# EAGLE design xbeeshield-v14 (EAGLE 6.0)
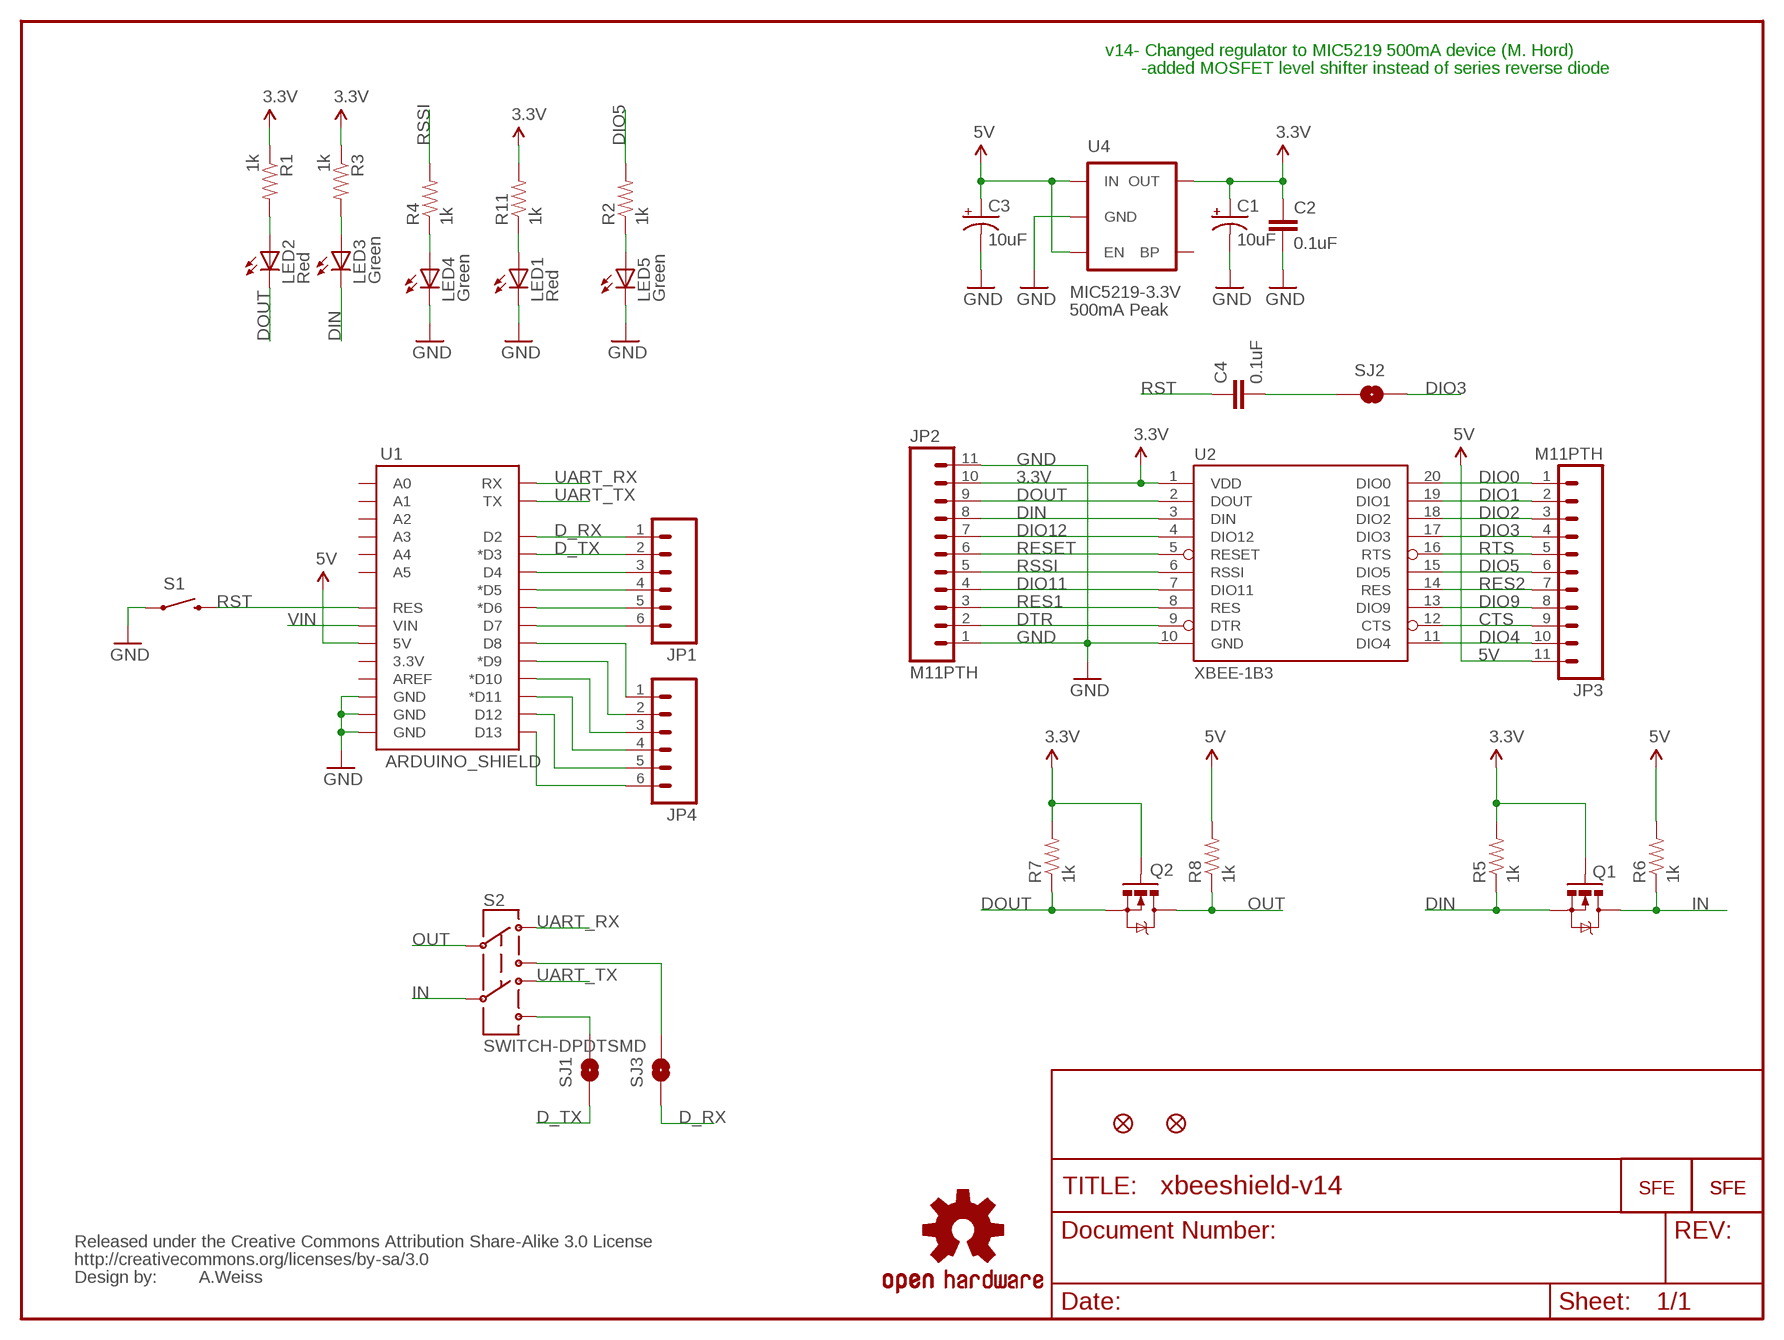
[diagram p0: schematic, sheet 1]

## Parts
C1  10uF  CAP_POL1206  [EIA3216]
C2  0.1uF  CAP0402-CAP  [0402-CAP]
C3  10uF  CAP_POL1206  [EIA3216]
C4  0.1uF  CAP0402-CAP  [0402-CAP]
JP1  M06SIP  [1X06]
JP2  M11PTH  [1X11]
JP3  M11PTH  [1X11]
JP4  M06SIP  [1X06]
JP5  FIDUCIAL1X2  [FIDUCIAL-1X2]
JP6  FIDUCIAL1X2  [FIDUCIAL-1X2]
JP7  LOGO-SFENEW  [SFE-NEW-WEBLOGO]
LED1  Red  LED0603  [LED-0603]
LED2  Red  LED0603  [LED-0603]
LED3  Green  LED0603  [LED-0603]
LED4  Green  LED0603  [LED-0603]
LED5  Green  LED0603  [LED-0603]
Q1  MOSFET-NCHANNELSMD  [SOT23-3]
Q2  MOSFET-NCHANNELSMD  [SOT23-3]
R1  1k  RESISTOR0402-RES  [0402-RES]
R2  1k  RESISTOR0402-RES  [0402-RES]
R3  1k  RESISTOR0402-RES  [0402-RES]
R4  1k  RESISTOR0402-RES  [0402-RES]
R5  1k  RESISTOR0402-RES  [0402-RES]
R6  1k  RESISTOR0402-RES  [0402-RES]
R7  1k  RESISTOR0402-RES  [0402-RES]
R8  1k  RESISTOR0402-RES  [0402-RES]
R11  1k  RESISTOR0402-RES  [0402-RES]
S1  SWITCH-MOMENTARY-2SMD  [TACTILE_SWITCH_SMD]
S2  SWITCH-DPDTSMD  [AYZ0202]
SJ1  D_TX  SOLDERJUMPERNC  [SJ_2S]
SJ2  SOLDERJUMPERTRACE  [SJ_2S-TRACE]
SJ3  D_RX  SOLDERJUMPERNC  [SJ_2S]
U1  ARDUINO_SHIELD  ARDUINO_SHIELDLABEL  [DUEMILANOVE_SHIELD]
U2  XBEE-1B3  [XBEE-SMD]
U4  V_REG_LDOSMD  [SOT23-5]
U$1  LOGO-SFESK  [SFE-LOGO-FLAME]
U$4  LOGO-SFENEW  [SFE-NEW-WEBLOGO]
U$5  CREATIVE_COMMONS  [CREATIVE_COMMONS]
U$8  OSHW-LOGOS  [OSHW-LOGO-S]

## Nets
3.3V: C1.A(+) C2.1 JP2.10 Q1.1(G) Q2.1(G) R1.1 R3.1 R5.2 R7.2 R11.2 U2.1(VDD) U4.5(OUT)
5V: C3.A(+) JP3.11 R6.2 R8.2 U1.5V U4.1(IN) U4.3(EN)
CTS: JP3.9 U2.12(CTS)
D_RX: JP1.1 SJ3.1 U1.D2
D_TX: JP1.2 SJ1.1 U1.D3(*D3)
DIN: JP2.8 LED3.C Q1.2(S) R5.1 U2.3(DIN)
DIO0: JP3.1 U2.20(DIO0)
DIO1: JP3.2 U2.19(DIO1)
DIO2: JP3.3 U2.18(DIO2)
DIO3: JP3.4 SJ2.2 U2.17(DIO3)
DIO4: JP3.10 U2.11(DIO4)
DIO5: JP3.6 R2.2 U2.15(DIO5)
DIO9: JP3.8 U2.13(DIO9)
DIO11: JP2.4 U2.7(DIO11)
DIO12: JP2.7 U2.4(DIO12)
DOUT: JP2.9 LED2.C Q2.2(S) R7.1 U2.2(DOUT)
DTR: JP2.2 U2.9(DTR)
GND: C1.C(-) C2.2 C3.C(-) JP2.1 JP2.11 LED1.C LED4.C LED5.C S1.1 U1.GND@0(GND) U1.GND@1(GND) U1.GND@2(GND) U2.10(GND) U4.2(GND)
IN: Q1.3(D) R6.1 S2.5
N$1: LED2.A R1.2
N$2: LED4.A R4.1
N$4: LED3.A R3.2
N$5: C4.2 SJ2.1
N$17: JP4.1 U1.D8
N$18: JP4.2 U1.D9(*D9)
N$30: JP4.3 U1.D10(*D10)
N$38: LED1.A R11.1
N$43: JP4.4 U1.D11(*D11)
N$55: JP4.5 U1.D12
N$67: JP4.6 U1.D13
N$139: LED5.A R2.1
N$140: S2.6 SJ1.2
N$141: S2.3 SJ3.2
N$142: JP1.3 U1.D4
N$143: JP1.4 U1.D5(*D5)
N$144: JP1.5 U1.D6(*D6)
N$145: JP1.6 U1.D7
OUT: Q2.3(D) R8.1 S2.2
RES1: JP2.3 U2.8(RES)
RES2: JP3.7 U2.14(RES)
RESET: JP2.6 U2.5(RESET)
RSSI: JP2.5 R4.2 U2.6(RSSI)
RST: C4.1 S1.3 U1.RES
RTS: JP3.5 U2.16(RTS)
UART_RX: S2.1 U1.RX
UART_TX: S2.4 U1.TX
VIN: U1.VIN
Unconnected: U1.3.3V U1.A0 U1.A1 U1.A2 U1.A3 U1.A4 U1.A5 U1.AREF U4.4(BP)

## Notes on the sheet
- v14- Changed regulator to MIC5219 500mA device (M. Hord)
- -added MOSFET level shifter instead of series reverse diode
- MIC5219-3.3V
- 500mA Peak
- A.Weiss

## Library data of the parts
C1 C3 = SparkFun:CAP_POL: Capacitor Polarized
C2 C4 = SparkFun:CAP: Capacitor
JP1 JP4 = SparkFun:M06: Header 6 Standard 6-pin 0.1" header. Use with straight break away headers (SKU : PRT-00116), right angle break away headers (PRT-00553), swiss pins (PRT-00743), machine pins (PRT-00117), and female headers (PRT-00115). Molex polarized connector foot print use with SKU : PRT-08094 with associated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
JP2 JP3 = SparkFun:M11: Header 11 Standard 11-pin 0.1" header. Use with straight break away headers (SKU : PRT-00116), right angle break away headers (PRT-00553), swiss pins (PRT-00743), machine pins (PRT-00117), and female headers (PRT-00115).
JP5 JP6 = SparkFun:FIDUCIAL: Fiducial Alignment Points
JP7 = SparkFun-Aesthetics:LOGO-SFE: Spark Fun Electronics PCB Logo
LED1-LED5 = SparkFun:LED: LEDs
Q1 Q2 = SparkFun-DiscreteSemi:MOSFET-NCHANNEL: Generic NMOS footprint
R1-R8 R11 = SparkFun:RESISTOR: Resistor
S1 = SparkFun:SWITCH-MOMENTARY-2
S2 = SparkFun:SWITCH-DPDT: DPDT Version of the COM-00597
SJ1-SJ3 = SparkFun:SOLDERJUMPER: Solder Jumper
U1 = SparkFun:ARDUINO_SHIELD
U2 = SparkFun:XBEE-1
U4 = SparkFun-PowerIC:V_REG_LDO: Voltage Regulator LDO Standard 150mA LDO voltage regulator in SOT-23 layout. Micrel part MIC5205. BP (by-pass) pin is used to lower output noise with 470pF cap.
U$1 U$4 = SparkFun:LOGO-SFE: Spark Fun Electronics PCB Logo
U$5 = SparkFun:CREATIVE_COMMONS
U$8 = SparkFun-Aesthetics:OSHW-LOGO: Open Source Hardware Logo This logo indicates the piece of hardware it is found on incorporates a OSHW license and/or adheres to the definition of open source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

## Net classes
0 default: width 0.203 mm
1 vcc: width 0.305 mm

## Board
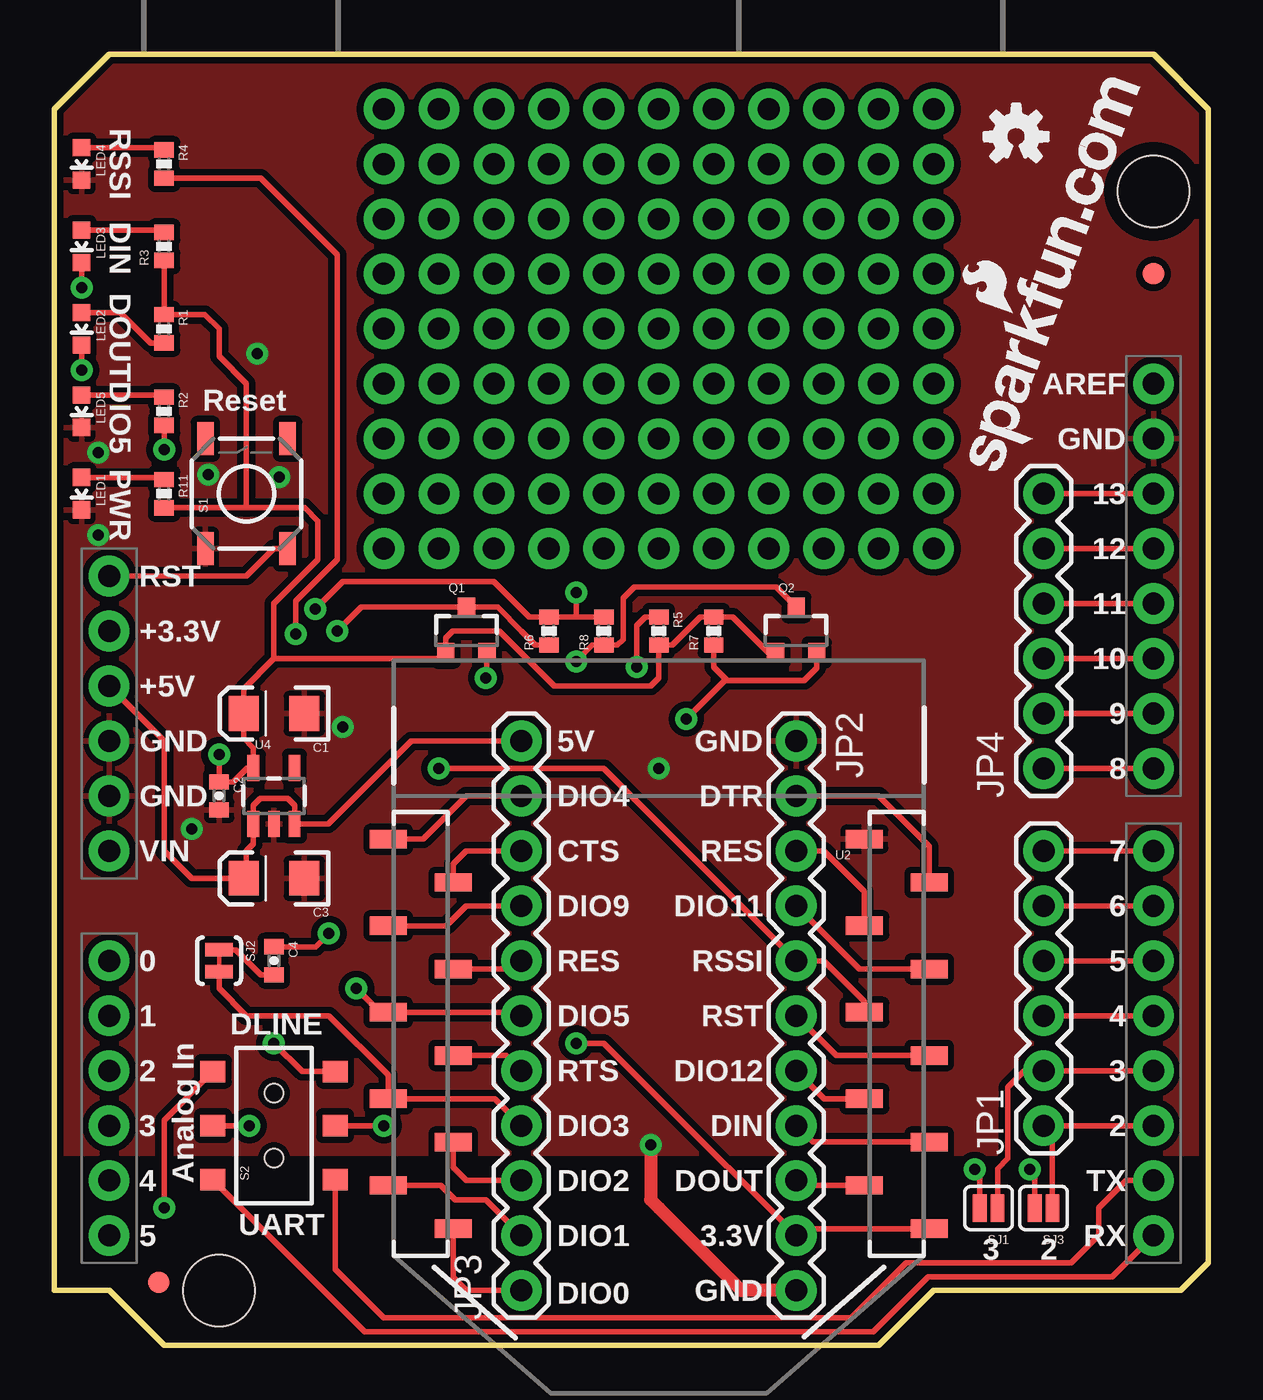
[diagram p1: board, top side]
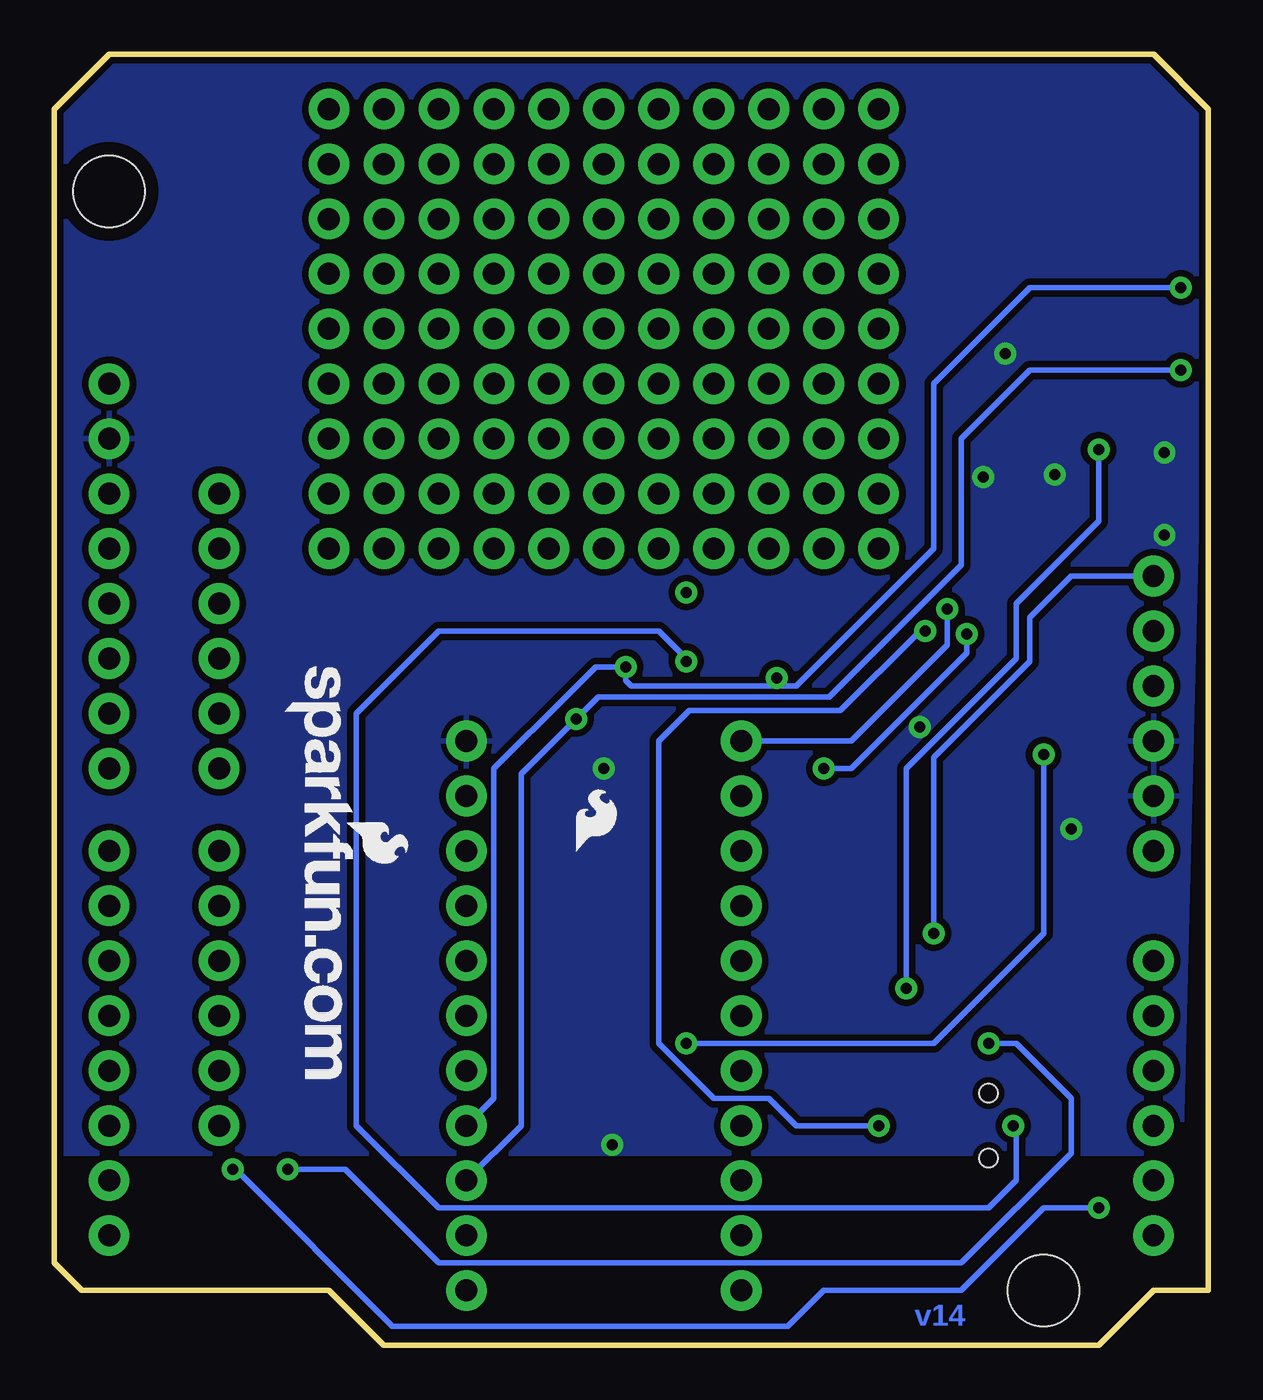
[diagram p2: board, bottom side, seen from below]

Size 53.34 x 59.69 mm. Coordinates in mm from the lower left corner, seen from the top.
Outline: 0,2.54 0,57.15 2.54,59.69 50.8,59.69 53.34,57.15 53.34,3.81 52.07,2.54 40.64,2.54 38.1,0 5.08,0 2.54,2.54 0,2.54
Copper layers (1*16): Top 0.035mm / dielectric 1.5mm / Bottom 0.035mm
Design rules: minimum track width 8mil, minimum drill 20mil, track to track 8mil, track to pad 8mil, pad to pad 8mil, via to via 8mil, smd to smd 8mil, copper to edge 8mil, drill to drill 8mil, minimum pad ring 12mil, minimum via ring 10mil, stop-mask expansion 4mil, vias tented up to drill 20mil, thermal gap 10mil

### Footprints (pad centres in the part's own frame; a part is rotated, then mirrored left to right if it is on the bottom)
EIA3216 = smd 1.4 x 1.6: A 1.4,0; C -1.4,0
0402-CAP = smd 0.7 x 0.9: 1 -0.65,0; 2 0.65,0
1X06 = drill 1.016 pad 1.88: 1 0,0; 2 2.54,0; 3 5.08,0; 4 7.62,0; 5 10.16,0; 6 12.7,0
1X11 = drill 1.016 pad 1.88: 1 0,0; 2 2.54,0; 3 5.08,0; 4 7.62,0; 5 10.16,0; 6 12.7,0; 7 15.24,0; 8 17.78,0; 9 20.32,0; 10 22.86,0; 11 25.4,0
FIDUCIAL-1X2 = smd 1 x 1: 1 0,0
LED-0603 = smd 0.8 x 0.8: A 0,-0.75; C 0,0.75
SOT23-3 = smd 0.8 x 0.9: 1 -0.95,-1; 2 0.95,-1; 3 0,1.1
0402-RES = smd 0.7 x 0.9: 1 -0.65,0; 2 0.65,0
TACTILE_SWITCH_SMD = smd 1.524 x 0.762: 1 -2.54,1.905; 2 2.54,1.905; 3 -2.54,-1.905; 4 2.54,-1.905
AYZ0202 = smd 1 x 1.15: 1 -2.5,2.825; 2 0,2.825; 3 2.5,2.825; 4 -2.5,-2.825; 5 0,-2.825; 6 2.5,-2.825 | hole 0.85: 1.5,0; -1.5,0
SJ_2S = smd 0.635 x 1.27: 1 -0.412,0; 2 0.412,0
SJ_2S-TRACE = smd 0.635 x 1.27: 1 -0.508,0; 2 0.508,0
DUEMILANOVE_SHIELD = drill 1.016 pad 1.88: 3.3V 50.8,26.67; 5V 50.8,29.21; A0 50.8,41.91; A1 50.8,44.45; A2 50.8,46.99; A3 50.8,49.53; A4 50.8,52.07; A5 50.8,54.61; AREF 2.54,15.24; D2 2.54,49.53; D3 2.54,46.99; D4 2.54,44.45; D5 2.54,41.91; D6 2.54,39.37; D7 2.54,36.83; D8 2.54,33.02; D9 2.54,30.48; D10 2.54,27.94; D11 2.54,25.4; D12 2.54,22.86; D13 2.54,20.32; GND@0 50.8,31.75; GND@1 50.8,34.29; GND@2 2.54,17.78; RES 50.8,24.13; RX 2.54,54.61; TX 2.54,52.07; VIN 50.8,36.83 | hole 3.302: 45.72,57.15; 2.54,6.35
XBEE-SMD = smd 1.7 x 0.85: 1 -12.5,20; 2 -9.5,18; 3 -12.5,16; 4 -9.5,14; 5 -12.5,12; 6 -9.5,10; 7 -12.5,8; 8 -9.5,6; 9 -12.5,4; 10 -9.5,2; 11 12.5,2; 12 9.5,4; 13 12.5,6; 14 9.5,8; 15 12.5,10; 16 9.5,12; 17 12.5,14; 18 9.5,16; 19 12.5,18; 20 9.5,20
SOT23-5 = smd 0.55 x 1.2: 1 -0.95,-1.3; 2 0,-1.3; 3 0.95,-1.3; 4 0.95,1.3; 5 -0.95,1.3

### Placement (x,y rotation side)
C1  10.16,29.21 180 top
C2  7.62,25.4 270 top
C3  10.16,21.59 180 top
C4  10.16,17.78 270 top
JP1  45.72,10.16 90 top
JP2  34.29,27.94 270 top
JP3  21.59,2.54 90 top
JP4  45.72,26.67 90 top
JP5  4.83,2.92 0 top
JP6  50.8,49.53 0 top
JP7  42.67,31.37 270 bottom
LED1  1.27,39.37 180 top
LED2  1.27,46.99 180 top
LED3  1.27,50.8 180 top
LED4  1.27,54.61 180 top
LED5  1.27,43.18 180 top
Q1  19.05,33.02 0 top
Q2  34.29,33.02 0 top
R1  5.08,46.99 270 top
R2  5.08,43.18 270 top
R3  5.08,50.8 90 top
R4  5.08,54.61 270 top
R5  27.94,33.02 270 top
R6  22.86,33.02 90 top
R7  30.48,33.02 90 top
R8  25.4,33.02 90 top
R11  5.08,39.37 270 top
S1  8.89,39.37 90 top
S2  10.16,10.16 90 top
SJ1  43.18,6.35 180 top
SJ2  7.62,17.78 270 top
SJ3  45.72,6.35 180 top
U1  53.34,59.69 180 top
U2  27.94,25.4 180 top
U4  10.16,25.4 0 top
U$1  29.21,22.86 0 bottom
U$4  44.54,39.97 70 top
U$5  not placed on the board
U$8  44.45,55.88 0 top

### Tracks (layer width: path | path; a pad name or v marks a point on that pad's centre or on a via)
3.3V  (via drill 0.51)
  Top 0.254: R3.1 R1.1 6.97,47.64 7.62,46.99 7.62,45.72 8.89,44.45 8.89,40.64 8.89,38.72 | U2.1 34.61,5.4 JP2.10 27.94,11.43 25.4,13.97 v24.13,13.97 | 10.16,31.75 8.76,30.35 C1.A 8.76,28.07 9.21,27.62 U4.5 8.92,26.7 8.27,26.05 C2.1 v7.62,27.3 | Q2.1 33,32.02 32,33.02 31.35,33.67 R7.2 29.86,33.67 29.21,33.02 28.56,32.37 R5.2 27.94,30.86 27.56,30.48 23.11,30.48 20.57,33.02 18.41,33.02 18.16,32.77 18.1,32.7 Q1.1 17.83,31.75 10.16,31.75 | R11.2 6.97,38.72 8.89,38.72 | 8.89,38.72 11.57,38.72 12.19,38.1 12.19,36.32 10.16,34.29 10.16,31.75
  Bottom 0.254: v24.13,13.97 12.7,13.97 7.62,19.05 v7.62,27.3
5V  (via drill 0.51)
  Top 0.254: U1.5V 5.08,27.94 5.08,22.86 6.35,21.59 C3.A 8.89,21.72 8.89,22.86 9.21,23.18 U4.1 9.21,24.96 9.53,25.27 10.79,25.27 11.11,24.96 U4.3 12.67,24.1 16.51,27.94 JP3.11 | 24.13,33.67 R6.2 21.96,33.67 20.32,35.31 14.1,35.31 13.34,35.31 v12.06,34.04 | 24.13,33.67 R8.2 | v24.13,34.8 24.13,33.67
  Bottom 0.254: JP3.11 16.51,27.94 12.7,31.75 12.06,32.38 v12.06,34.04
CTS
  Top 0.254: U2.12 18.44,22.25 19.05,22.86 JP3.9
D_RX
  Top 0.254: U1.D2 JP1.1 46.13,9.75 SJ3.1
D_TX
  Top 0.254: U1.D3 JP1.2 44.83,12.7 44.07,11.94 44.07,8.64 43.59,8.16 SJ1.1
DIN  (via drill 0.51)
  Top 0.254: v1.27,48.9 LED3.C | R5.1 27.32,33.67 26.92,33.27 v26.92,31.37 | Q1.2 20,30.92 v19.94,30.86 | U2.3 35.05,9.4 JP2.8
  Bottom 0.254: v1.27,48.9 3.17,48.9 8.26,48.9 12.7,44.45 12.7,40.64 12.7,38.1 12.7,36.83 19.05,30.48 19.94,30.48 | JP2.8 33.02,11.43 33.02,26.67 29.59,30.1 28.32,31.37 v26.92,31.37 26.92,30.73 26.67,30.48 19.94,30.48 | v19.94,30.86 19.94,30.48
DIO0
  Top 0.254: U2.20 18.44,3.15 19.05,2.54 JP3.1
DIO1
  Top 0.254: JP3.2 19.94,6.73 18.54,6.73 17.87,7.4 U2.19
DIO2
  Top 0.254: U2.18 18.44,8.23 19.05,7.62 JP3.3
DIO3
  Top 0.254: JP3.4 20.35,11.4 U2.17 15.44,12.5 12.7,15.24 8.89,15.24 7.62,16.51 SJ2.2
DIO4
  Top 0.254: U2.11 17.05,23.4 19.05,25.4 JP3.10
DIO5  (via drill 0.51)
  Top 0.254: v5.08,41.4 R2.2 | JP3.6 21.43,15.4 U2.15 15.08,15.4 v13.97,16.51
  Bottom 0.254: v13.97,16.51 13.97,25.4 13.97,26.67 8.89,31.75 8.89,34.29 5.08,38.1 v5.08,41.4
DIO9
  Top 0.254: U2.13 18.13,19.4 19.05,20.32 JP3.8
DIO11
  Top 0.254: U2.7 37.21,17.4 JP2.4
DIO12
  Top 0.254: U2.4 35.59,11.4 JP2.7
DOUT  (via drill 0.51)
  Top 0.254: v1.27,45.09 LED2.C | Q2.2 35.24,31.3 34.67,30.73 31.11,30.73 | 31.11,30.73 30.48,31.37 R7.1 | 31.11,30.73 30.99,30.73 v29.21,28.96 | U2.2 34.51,7.4 JP2.9
  Bottom 0.254: v1.27,45.09 4.45,45.09 8.26,45.09 11.43,41.91 11.43,39.37 11.43,36.07 17.53,29.97 28.19,29.97 v29.21,28.96 31.75,26.42 31.75,10.16 JP2.9
DTR
  Top 0.254: JP2.2 38.1,25.4 40.44,23.06 U2.9
GND  (via drill 0.51)
  Top 0.61: JP2.11 31.75,2.54 27.94,6.35 27.56,6.73 v27.56,9.27
  other vias: 2.03,37.47 6.35,23.88 13.34,28.57 9.4,45.85 27.94,26.67 2.03,41.27 7.11,40.26 10.41,40.13
  pour Top (isolate 0.305): 0,8.89 0,59.69 53.34,59.69 53.34,8.89
  pour Bottom (isolate 0.305): 0,59.69 1.27,8.89 54.61,8.89 53.34,59.69
IN  (via drill 0.51)
  Top 0.254: R6.1 22.24,32.37 21.59,33.02 20.49,34.12 Q1.3 14.18,34.12 v13.08,33.02 | S2.5 v15.24,10.16
  Bottom 0.254: v15.24,10.16 19.05,10.16 20.32,11.43 22.86,11.43 25.4,13.97 25.4,27.94 24,29.34 17.02,29.34 13.46,32.89 13.21,32.89 v13.08,33.02
N$1
  Top 0.254: LED2.A 3.06,47.74 4.46,46.34 R1.2
N$2
  Top 0.254: LED4.A 4.98,55.36 R4.1
N$4
  Top 0.254: LED3.A 4.98,51.55 R3.2
N$5
  Top 0.254: C4.2 9.54,17.13 8.38,18.29 SJ2.1
N$17
  Top 0.254: JP4.1 U1.D8
N$18
  Top 0.254: JP4.2 U1.D9
N$30
  Top 0.254: JP4.3 U1.D10
N$31  (via drill 1.02 pad 1.88)
  other vias: 40.64,36.83
N$32  (via drill 1.02 pad 1.88)
  other vias: 38.1,36.83
N$33  (via drill 1.02 pad 1.88)
  other vias: 35.56,36.83
N$34  (via drill 1.02 pad 1.88)
  other vias: 33.02,36.83
N$35  (via drill 1.02 pad 1.88)
  other vias: 30.48,36.83
N$36  (via drill 1.02 pad 1.88)
  other vias: 27.94,36.83
N$37  (via drill 1.02 pad 1.88)
  other vias: 25.4,36.83
N$38
  Top 0.254: LED1.A 4.98,40.12 R11.1
N$39  (via drill 1.02 pad 1.88)
  other vias: 22.86,36.83
N$40  (via drill 1.02 pad 1.88)
  other vias: 20.32,36.83
N$41  (via drill 1.02 pad 1.88)
  other vias: 17.78,36.83
N$42  (via drill 1.02 pad 1.88)
  other vias: 15.24,36.83
N$43
  Top 0.254: JP4.4 U1.D11
N$44  (via drill 1.02 pad 1.88)
  other vias: 40.64,39.37
N$45  (via drill 1.02 pad 1.88)
  other vias: 38.1,39.37
N$46  (via drill 1.02 pad 1.88)
  other vias: 35.56,39.37
N$47  (via drill 1.02 pad 1.88)
  other vias: 33.02,39.37
N$48  (via drill 1.02 pad 1.88)
  other vias: 30.48,39.37
N$49  (via drill 1.02 pad 1.88)
  other vias: 27.94,39.37
N$50  (via drill 1.02 pad 1.88)
  other vias: 25.4,39.37
N$51  (via drill 1.02 pad 1.88)
  other vias: 22.86,39.37
N$52  (via drill 1.02 pad 1.88)
  other vias: 20.32,39.37
N$53  (via drill 1.02 pad 1.88)
  other vias: 17.78,39.37
N$54  (via drill 1.02 pad 1.88)
  other vias: 15.24,39.37
N$55
  Top 0.254: JP4.5 U1.D12
N$56  (via drill 1.02 pad 1.88)
  other vias: 40.64,41.91
N$57  (via drill 1.02 pad 1.88)
  other vias: 38.1,41.91
N$58  (via drill 1.02 pad 1.88)
  other vias: 35.56,41.91
N$59  (via drill 1.02 pad 1.88)
  other vias: 33.02,41.91
N$60  (via drill 1.02 pad 1.88)
  other vias: 30.48,41.91
N$61  (via drill 1.02 pad 1.88)
  other vias: 27.94,41.91
N$62  (via drill 1.02 pad 1.88)
  other vias: 25.4,41.91
N$63  (via drill 1.02 pad 1.88)
  other vias: 22.86,41.91
N$64  (via drill 1.02 pad 1.88)
  other vias: 20.32,41.91
N$65  (via drill 1.02 pad 1.88)
  other vias: 17.78,41.91
N$66  (via drill 1.02 pad 1.88)
  other vias: 15.24,41.91
N$67
  Top 0.254: JP4.6 U1.D13
N$68  (via drill 1.02 pad 1.88)
  other vias: 40.64,44.45
N$69  (via drill 1.02 pad 1.88)
  other vias: 38.1,44.45
N$70  (via drill 1.02 pad 1.88)
  other vias: 35.56,44.45
N$71  (via drill 1.02 pad 1.88)
  other vias: 33.02,44.45
N$72  (via drill 1.02 pad 1.88)
  other vias: 30.48,44.45
N$73  (via drill 1.02 pad 1.88)
  other vias: 27.94,44.45
N$74  (via drill 1.02 pad 1.88)
  other vias: 25.4,44.45
N$75  (via drill 1.02 pad 1.88)
  other vias: 22.86,44.45
N$76  (via drill 1.02 pad 1.88)
  other vias: 20.32,44.45
N$77  (via drill 1.02 pad 1.88)
  other vias: 17.78,44.45
N$78  (via drill 1.02 pad 1.88)
  other vias: 15.24,44.45
N$80  (via drill 1.02 pad 1.88)
  other vias: 40.64,46.99
N$81  (via drill 1.02 pad 1.88)
  other vias: 38.1,46.99
N$82  (via drill 1.02 pad 1.88)
  other vias: 35.56,46.99
N$83  (via drill 1.02 pad 1.88)
  other vias: 33.02,46.99
N$84  (via drill 1.02 pad 1.88)
  other vias: 30.48,46.99
N$85  (via drill 1.02 pad 1.88)
  other vias: 27.94,46.99
N$86  (via drill 1.02 pad 1.88)
  other vias: 25.4,46.99
N$87  (via drill 1.02 pad 1.88)
  other vias: 22.86,46.99
N$88  (via drill 1.02 pad 1.88)
  other vias: 20.32,46.99
N$89  (via drill 1.02 pad 1.88)
  other vias: 17.78,46.99
N$90  (via drill 1.02 pad 1.88)
  other vias: 15.24,46.99
N$92  (via drill 1.02 pad 1.88)
  other vias: 40.64,49.53
N$93  (via drill 1.02 pad 1.88)
  other vias: 38.1,49.53
N$94  (via drill 1.02 pad 1.88)
  other vias: 35.56,49.53
N$95  (via drill 1.02 pad 1.88)
  other vias: 33.02,49.53
N$96  (via drill 1.02 pad 1.88)
  other vias: 30.48,49.53
N$97  (via drill 1.02 pad 1.88)
  other vias: 27.94,49.53
N$98  (via drill 1.02 pad 1.88)
  other vias: 25.4,49.53
N$99  (via drill 1.02 pad 1.88)
  other vias: 22.86,49.53
N$100  (via drill 1.02 pad 1.88)
  other vias: 20.32,49.53
N$101  (via drill 1.02 pad 1.88)
  other vias: 17.78,49.53
N$102  (via drill 1.02 pad 1.88)
  other vias: 15.24,49.53
N$104  (via drill 1.02 pad 1.88)
  other vias: 40.64,52.07
N$105  (via drill 1.02 pad 1.88)
  other vias: 38.1,52.07
N$106  (via drill 1.02 pad 1.88)
  other vias: 35.56,52.07
N$107  (via drill 1.02 pad 1.88)
  other vias: 33.02,52.07
N$108  (via drill 1.02 pad 1.88)
  other vias: 30.48,52.07
N$109  (via drill 1.02 pad 1.88)
  other vias: 27.94,52.07
N$110  (via drill 1.02 pad 1.88)
  other vias: 25.4,52.07
N$111  (via drill 1.02 pad 1.88)
  other vias: 22.86,52.07
N$112  (via drill 1.02 pad 1.88)
  other vias: 20.32,52.07
N$113  (via drill 1.02 pad 1.88)
  other vias: 17.78,52.07
N$114  (via drill 1.02 pad 1.88)
  other vias: 15.24,52.07
N$116  (via drill 1.02 pad 1.88)
  other vias: 40.64,54.61
N$117  (via drill 1.02 pad 1.88)
  other vias: 38.1,54.61
N$118  (via drill 1.02 pad 1.88)
  other vias: 35.56,54.61
N$119  (via drill 1.02 pad 1.88)
  other vias: 33.02,54.61
N$120  (via drill 1.02 pad 1.88)
  other vias: 30.48,54.61
N$121  (via drill 1.02 pad 1.88)
  other vias: 27.94,54.61
N$122  (via drill 1.02 pad 1.88)
  other vias: 25.4,54.61
N$123  (via drill 1.02 pad 1.88)
  other vias: 22.86,54.61
N$124  (via drill 1.02 pad 1.88)
  other vias: 20.32,54.61
N$125  (via drill 1.02 pad 1.88)
  other vias: 17.78,54.61
N$126  (via drill 1.02 pad 1.88)
  other vias: 15.24,54.61
N$128  (via drill 1.02 pad 1.88)
  other vias: 40.64,57.15
N$129  (via drill 1.02 pad 1.88)
  other vias: 38.1,57.15
N$130  (via drill 1.02 pad 1.88)
  other vias: 35.56,57.15
N$131  (via drill 1.02 pad 1.88)
  other vias: 33.02,57.15
N$132  (via drill 1.02 pad 1.88)
  other vias: 30.48,57.15
N$133  (via drill 1.02 pad 1.88)
  other vias: 27.94,57.15
N$134  (via drill 1.02 pad 1.88)
  other vias: 25.4,57.15
N$135  (via drill 1.02 pad 1.88)
  other vias: 22.86,57.15
N$136  (via drill 1.02 pad 1.88)
  other vias: 20.32,57.15
N$137  (via drill 1.02 pad 1.88)
  other vias: 17.78,57.15
N$138  (via drill 1.02 pad 1.88)
  other vias: 15.24,57.15
N$139
  Top 0.254: LED5.A 4.98,43.93 R2.1
N$140  (via drill 0.51)
  Top 0.254: v42.55,8.13 42.77,7.91 SJ1.2 | S2.6 11.47,12.66 v10.16,13.97
  Bottom 0.254: v42.55,8.13 39.88,8.13 35.56,3.81 11.43,3.81 6.35,8.89 6.35,11.43 8.89,13.97 v10.16,13.97
N$141  (via drill 0.51)
  Top 0.254: v45.09,8.13 45.31,7.91 SJ3.2 | v5.08,6.35 5.08,10.4 S2.3
  Bottom 0.254: v45.09,8.13 44.96,8.13 37.72,0.89 19.43,0.89 17.78,2.54 11.43,2.54 7.62,6.35 v5.08,6.35
N$142
  Top 0.254: JP1.3 U1.D4
N$143
  Top 0.254: JP1.4 U1.D5
N$144
  Top 0.254: JP1.5 U1.D6
N$145
  Top 0.254: JP1.6 U1.D7
OUT  (via drill 0.51)
  Top 0.254: Q2.3 33.36,35.05 27.43,35.05 26.8,35.05 26.67,34.92 26.29,34.54 26.29,32.64 26.02,32.37 R8.1 24.88,32.37 v24.13,31.62 | S2.2 7.62,10.16 v9.02,10.16
  Bottom 0.254: v24.13,31.62 24.13,31.75 25.4,33.02 35.56,33.02 39.37,29.21 39.37,10.16 35.56,6.35 11.43,6.35 10.16,6.35 8.89,7.62 8.89,10.03 v9.02,10.16
RES1
  Top 0.254: JP2.3 35.56,22.86 37.44,20.98 U2.8
RES2
  Top 0.254: U2.14 21.21,17.4 JP3.7
RESET
  Top 0.254: U2.5 36.13,13.4 JP2.6
RSSI  (via drill 0.51)
  Top 0.254: U2.6 37.44,15.9 35.56,17.78 JP2.5 25.4,26.67 v17.78,26.67 | v11.18,32.89 11.18,34.42 13.08,36.32 13.08,49.78 13.08,50.42 12.7,50.8 9.54,53.96 R4.2
  Bottom 0.254: v17.78,26.67 16.51,26.67 11.43,31.75 11.18,32 v11.18,32.89
RST  (via drill 0.51)
  Top 0.254: C4.1 12.08,18.43 v12.7,19.05 | U1.RES 7.62,35.56 8.89,35.56 10.16,36.83 S1.3
  Bottom 0.254: v12.7,19.05 12.7,25.4 12.7,27.18 8.26,31.62 8.26,33.66 6.35,35.56 U1.RES 4.32,35.56
RTS
  Top 0.254: U2.16 20.89,13.4 JP3.5
UART_RX
  Top 0.254: U1.RX 48.9,3.17 40.39,3.17 37.85,0.64 14.36,0.64 S2.1
UART_TX
  Top 0.254: S2.4 12.98,3.52 15.24,1.27 36.83,1.27 39.37,3.81 46.99,3.81 48.26,5.08 48.26,6.35 49.53,7.62 U1.TX

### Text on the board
Bottom: v14
tPlace: RSSI | DIN | DOUT | DIO5 | Reset | PWR | GND | 5V | DTR | DIO4 | RES | CTS | DIO11 | DIO9 | RSSI | RES | RST | DIO5 | DLINE | DIO12 | RTS | DIN | DIO3 | DOUT | DIO2 | 3.3V | UART | DIO1 | 3 | 2 | GND | DIO0
Reference: RSSI | DIN | DOUT | PWR | DIO5 | Reset | GND | 5V | DTR | DIO4 | RES | CTS | DIO11 | DIO9 | RSSI | RES | RST | DIO5 | DLINE | DIO12 | RTS | DIN | DIO3 | DOUT | DIO2 | 3.3V | UART | DIO1 | 3 | 2 | GND | DIO0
